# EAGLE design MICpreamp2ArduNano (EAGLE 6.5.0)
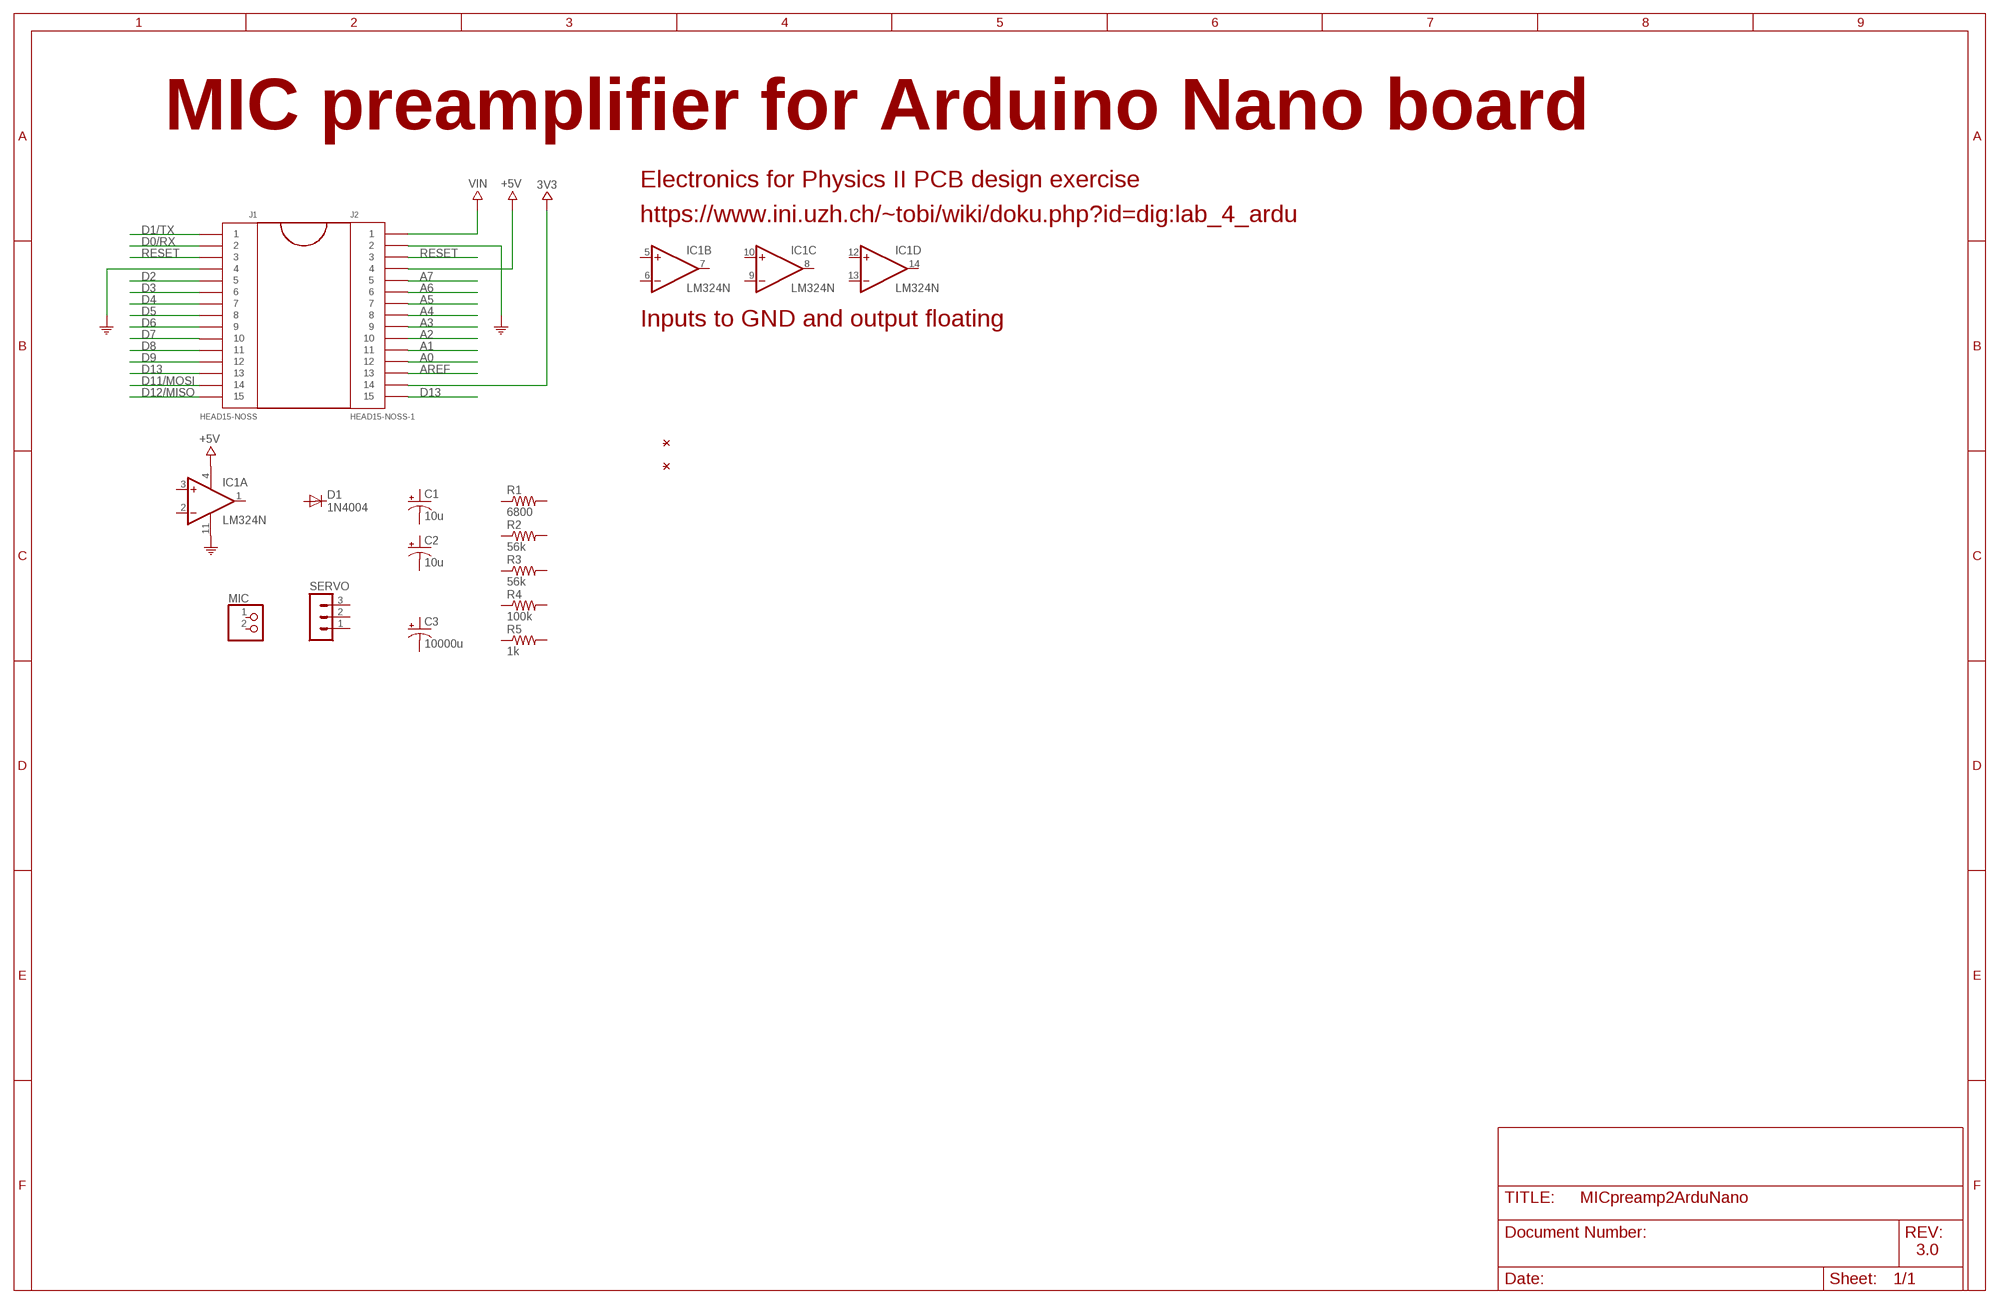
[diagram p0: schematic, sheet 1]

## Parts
C1  10u  CPOL-USE2.5-7  [E2,5-7]
C2  10u  CPOL-USE2.5-7  [E2,5-7]
C3  10000u  CPOL-USE10-20  [EB20D]
D1  1N4004  [DO41-10]
IC1  LM324N  [DIL14]
J1  HEAD15-NOSS  [HEAD15-NOSS]
J2  HEAD15-NOSS-1  [HEAD15-NOSS-1]
MIC  PINHD-1X2  [1X02]
R1  6800  R-US_0207/10  [0207/10]
R2  56k  R-US_0207/10  [0207/10]
R3  56k  R-US_0207/10  [0207/10]
R4  100k  R-US_0207/10  [0207/10]
R5  1k  R-US_0207/10  [0207/10]
SERVO  MA03-1  [MA03-1]

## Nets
3V3: J2.14
+5V: IC1.4(P:V+) J2.4
A0: J2.12
A1: J2.11
A2: J2.10
A3: J2.9
A4: J2.8
A5: J2.7
A6: J2.6
A7: J2.5
AREF: J2.13
COM: IC1.11(P:V-) J1.4 J2.2
D0/RX: J1.2
D1/TX: J1.1
D2: J1.5
D3: J1.6
D4: J1.7
D5: J1.8
D6: J1.9
D7: J1.10
D8: J1.11
D9: J1.12
D11/MOSI: J1.14
D12/MISO: J1.15
D13: J1.13
RESET: J1.3 J2.3
VIN: J2.1
Unconnected: C1.+ C1.- C2.+ C2.- C3.+ C3.- D1.A D1.C IC1.1(A:OUT) IC1.2(A:-IN) IC1.3(A:+IN) IC1.5(B:+IN) IC1.6(B:-IN) IC1.7(B:OUT) IC1.8(C:OUT) IC1.9(C:-IN) IC1.10(C:+IN) IC1.12(D:+IN) IC1.13(D:-IN) IC1.14(D:OUT) J2.15 MIC.1 MIC.2 R1.1 R1.2 R2.1 R2.2 R3.1 R3.2 R4.1 R4.2 R5.1 R5.2 SERVO.1 SERVO.2 SERVO.3

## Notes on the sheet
- MIC preamplifier for Arduino Nano board
- Electronics for Physics II PCB design exercise
- https://www.ini.uzh.ch/~tobi/wiki/doku.php?id=dig:lab_4_ardu
- Inputs to GND and output floating
- 3.0

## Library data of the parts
C1-C3 = resistor:CPOL-US: POLARIZED CAPACITOR, American symbol
D1 = diode:1N4004: DIODE
IC1 = linear:LM324: OP AMP
J1 = MyCON2:HEAD15-NOSS
J2 = MyCON2:HEAD15-NOSS-1
MIC = pinhead:PINHD-1X2: PIN HEADER
R1-R5 = resistor:R-US_: RESISTOR, American symbol
SERVO = con-lstb:MA03-1: PIN HEADER; OC_FARNELL: unknown; OC_NEWARK: unknown

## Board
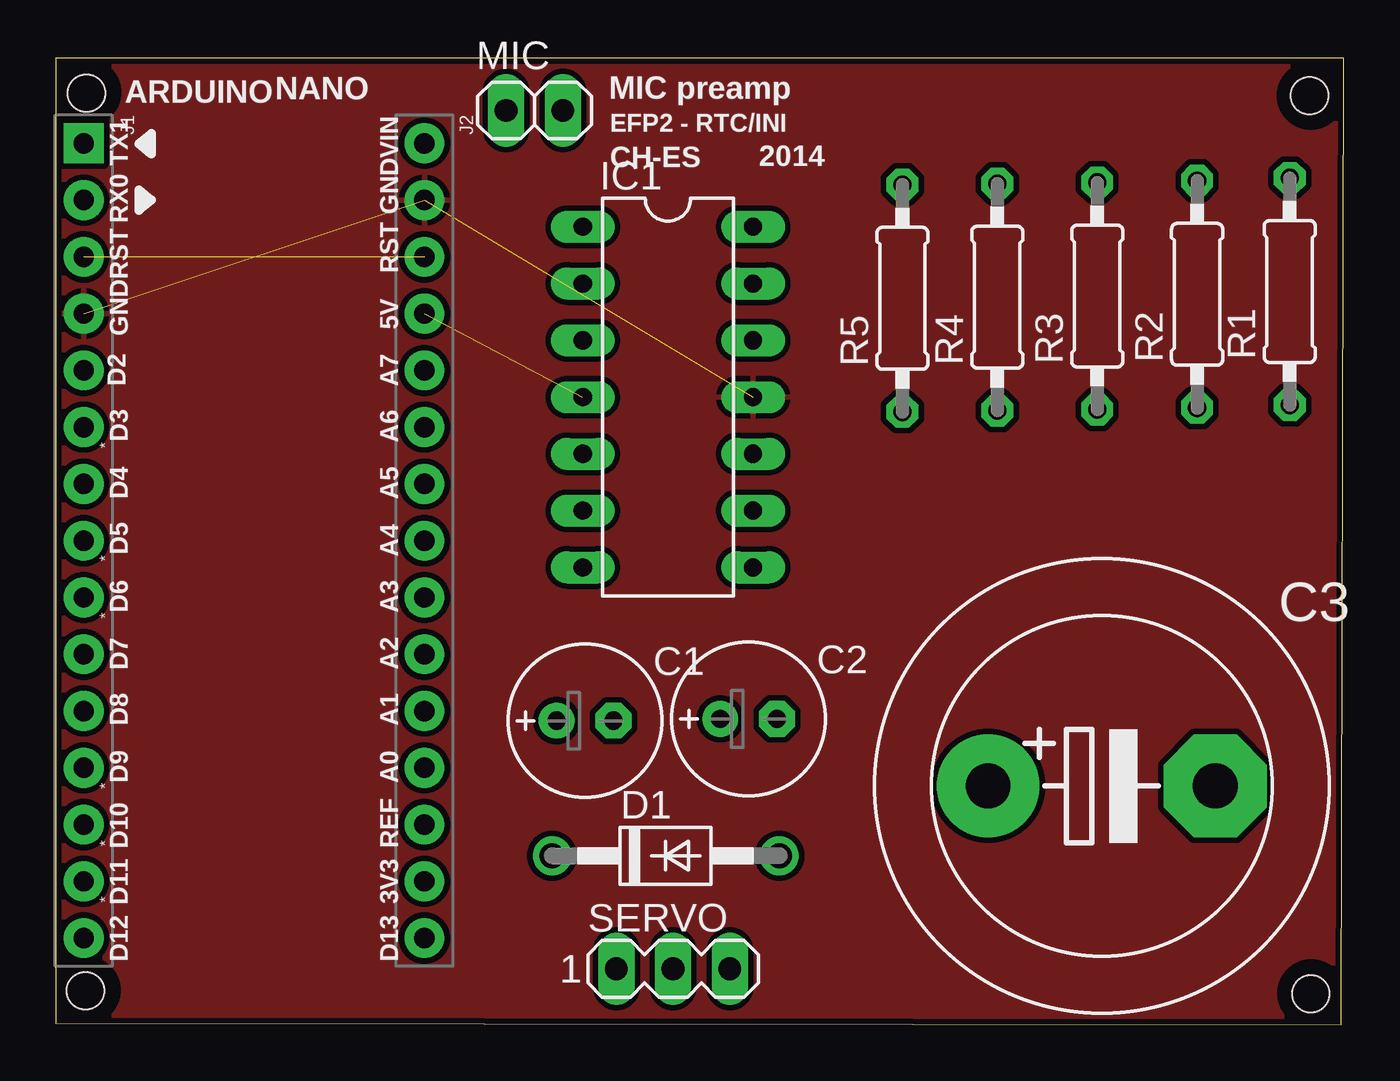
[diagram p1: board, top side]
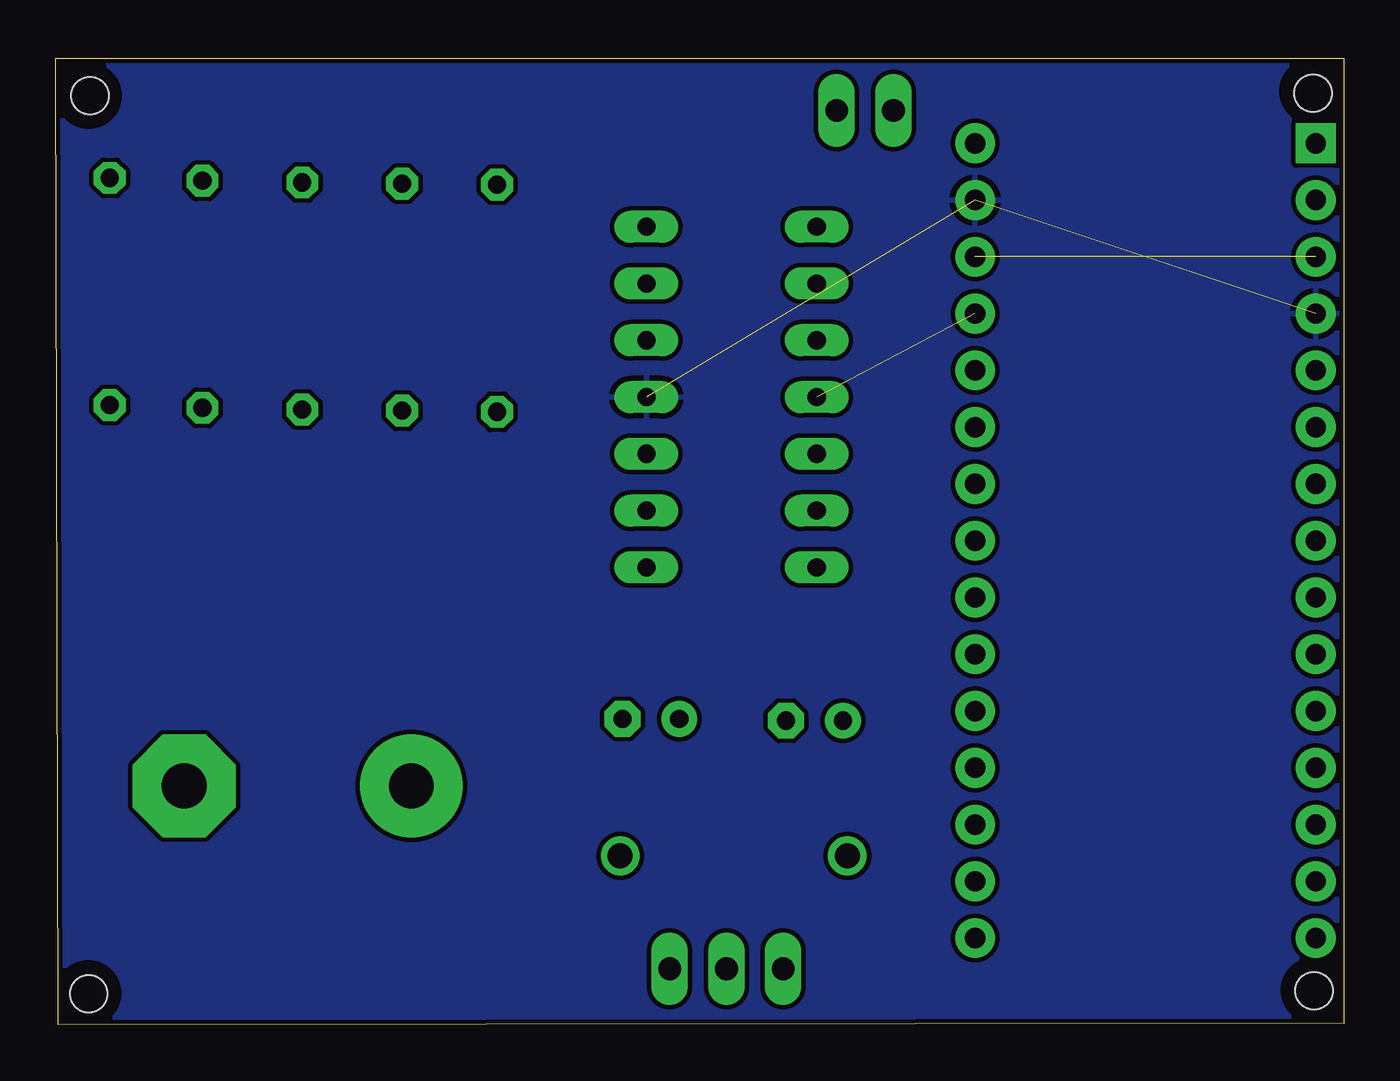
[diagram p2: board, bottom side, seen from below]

Size 57.61 x 43.26 mm. Coordinates in mm from the lower left corner, seen from the top.
Outline: 0,0.08 57.51,0 57.61,43.26 0,43.26 0,0.08
Copper layers (1*16): Top 0.035mm / dielectric 1.5mm / Bottom 0.035mm
Design rules "default *": minimum track width 8mil, minimum drill 16mil, track to track 8mil, track to pad 8mil, pad to pad 8mil, via to via 8mil, smd to smd 8mil, copper to edge 8mil, drill to drill 8mil, minimum pad ring 12mil, minimum via ring 8mil, stop-mask expansion 4mil, vias tented up to drill 18mil, thermal gap 10mil
Holes 1.65 mm at 1.32,1.52 56.13,1.4 56.08,41.58 1.37,41.68
tRestrict: area 0.2,0.4 to 2.5,2.7; area 55,40.4 to 57.3,42.7; area 55,0.3 to 57.3,2.6; area 0.3,40.6 to 2.5,42.9
bRestrict: area 55,0.3 to 57.3,2.6; area 0.2,0.4 to 2.5,2.7; area 0.3,40.6 to 2.5,42.9; area 55,40.4 to 57.3,42.7

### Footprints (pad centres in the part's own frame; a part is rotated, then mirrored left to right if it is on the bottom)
E2,5-7 = drill 0.813 pad 1.6: + -1.27,0 | drill 0.813 pad 1.6 octagon: - 1.27,0
EB20D = drill 2.007 pad 4.597: + -5.08,0 | drill 2.007 pad 4.597 octagon: - 5.08,0
DO41-10 = drill 1.118: A 5.08,0; C -5.08,0
DIL14 = drill 0.813 long: 1 -7.62,-3.81; 2 -5.08,-3.81; 3 -2.54,-3.81; 4 0,-3.81; 5 2.54,-3.81; 6 5.08,-3.81; 7 7.62,-3.81; 8 7.62,3.81; 9 5.08,3.81; 10 2.54,3.81; 11 0,3.81; 12 -2.54,3.81; 13 -5.08,3.81; 14 -7.62,3.81
HEAD15-NOSS = drill 0.914 pad 1.778 square: 1 0,0 | drill 0.914 pad 1.778: 2 2.54,0; 3 5.08,0; 4 7.62,0; 5 10.16,0; 6 12.7,0; 7 15.24,0; 8 17.78,0; 9 20.32,0; 10 22.86,0; 11 25.4,0; 12 27.94,0; 13 30.48,0; 14 33.02,0; 15 35.56,0
HEAD15-NOSS-1 = drill 0.914 pad 1.778: 1 0,0; 2 2.54,0; 3 5.08,0; 4 7.62,0; 5 10.16,0; 6 12.7,0; 7 15.24,0; 8 17.78,0; 9 20.32,0; 10 22.86,0; 11 25.4,0; 12 27.94,0; 13 30.48,0; 14 33.02,0; 15 35.56,0
1X02 = drill 1.016 long: 1 -1.27,0; 2 1.27,0
0207/10 = drill 0.813 octagon: 1 -5.08,0; 2 5.08,0
MA03-1 = drill 1.016 long: 1 -2.54,0; 2 0,0; 3 2.54,0

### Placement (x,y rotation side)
C1  23.67,13.61 0 top
C2  30.99,13.69 0 top
C3  46.79,10.69 0 top
D1  27.28,7.57 0 top
IC1  27.38,28.09 270 top
J1  1.24,39.45 270 top
J2  16.48,39.45 270 top
MIC  21.41,40.92 0 top
R1  55.19,32.82 90 top
R2  51.05,32.69 90 top
R3  46.58,32.61 90 top
R4  42.11,32.56 90 top
R5  37.87,32.51 90 top
SERVO  27.61,2.51 0 top

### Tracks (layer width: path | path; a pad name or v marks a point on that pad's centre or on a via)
+5V  (1 unrouted)
COM  (2 unrouted)
  pour Top (isolate 0.254): -0.03,0.1 -0.05,43 57.53,43 57.43,0.05
  pour Bottom (isolate 0.203): -0.03,0.1 -0.05,43.03 57.61,42.98 57.4,0.05
RESET  (1 unrouted)

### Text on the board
tPlace: ARDUINO | NANO | MIC preamp | EFP2 - RTC/INI | VIN | TX1 | CH-ES | 2014 | RX0 | GND | RST | RST | GND | 5V | D2 | A7 | * | D3 | A6 | D4 | A5 | * | D5 | A4 | * | D6 | A3 | D7 | A2 | D8 | A1 | D9 | A0 | * | * | D10 | REF | * | D11 | 3V3 | D12 | D13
